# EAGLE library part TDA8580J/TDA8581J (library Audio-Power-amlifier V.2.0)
The TDA8580J is a stereo Bridge-Tied Load (BTL) or a quad Single-Ended (SE) amplifier that operates over a wide supply voltage range from 8 to 24 V. This makes it suitable for applications such as television, home-sound systems and active speakers. The TDA8581 is a stereo bridge-tied load (BTL) or a quad single-ended amplifier that operates over a wide supply voltage range from 8 to 28 V. This makes it suitable for many applications, such as car radios, television and home-sound systems.
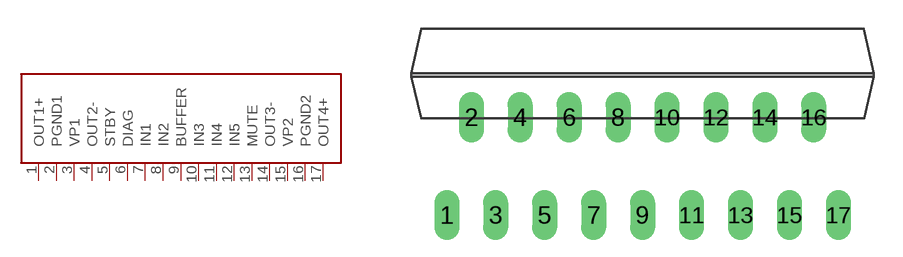
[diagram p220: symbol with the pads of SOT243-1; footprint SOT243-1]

Designator prefix IC

## TDA8580J/TDA8581J  [SOT243-1]
1  OUT1+  out
2  PGND1  pwr
3  VP1  pwr
4  OUT2-  out
5  STBY  in
6  DIAG  out
7  IN1  in
8  IN2  in
9  BUFFER  out
10  IN3  in
11  IN4  in
12  IN5  in
13  MUTE  in
14  OUT3-  out
15  VP2  pwr
16  PGND2  pwr
17  OUT4+  out

## Footprint SOT243-1 (pad centres in mm)
DBS17P: plastic DIL-bent-SIL power package; 17 leads (lead length 7.7 mm)
drill 0.8 long: 1 -10.16,-5.08; 2 -8.89,0; 3 -7.62,-5.08; 4 -6.35,0; 5 -5.08,-5.08; 6 -3.81,0; 7 -2.54,-5.08; 8 -1.27,0; 9 0,-5.08; 10 1.27,0; 11 2.54,-5.08; 12 3.81,0; 13 5.08,-5.08; 14 6.35,0; 15 7.62,-5.08; 16 8.89,0; 17 10.17,-5.08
